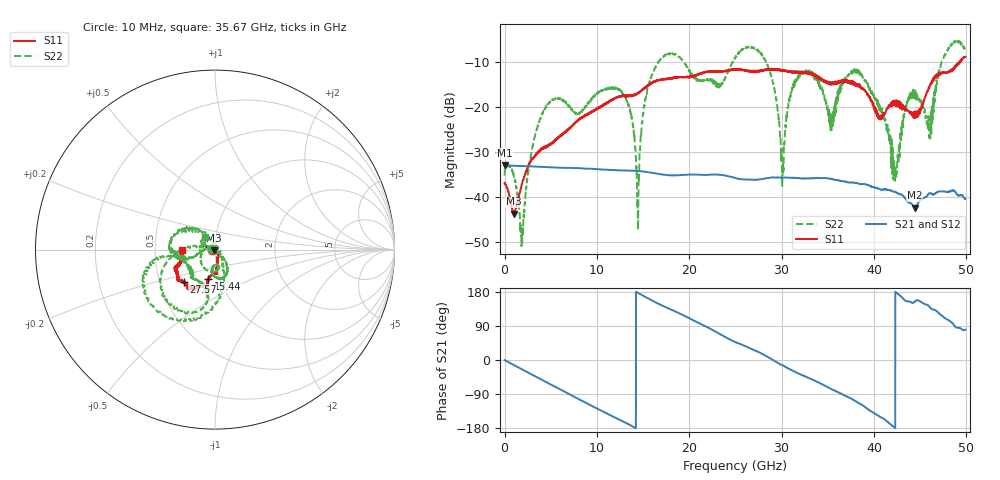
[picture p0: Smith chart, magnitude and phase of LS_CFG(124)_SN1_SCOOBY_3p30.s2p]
!Keysight Technologies,N5245B,MY58422026,A.13.80.08
!Date: Friday, March 20, 2020 00:06:09
!Correction: S11(Full 2 Port(1,2))
!S21(Full 2 Port(1,2))
!S12(Full 2 Port(1,2))
!S22(Full 2 Port(1,2))
!S2P File: Measurements: S11, S21, S12, S22:
# Hz S DB R 50.0
!freq dBS11 angS11 dBS21 angS21 dBS12 angS12 dBS22 angS22
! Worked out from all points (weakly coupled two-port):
!   4991 points, 10 MHz to 49.91 GHz, reference 50 ohm
!   highest |S21| = -32.99 dB at 10 MHz (marker M1); lowest = -42.5 dB at 44.42 GHz (marker M2)
!   lowest |S11| = -43.8 dB at 990 MHz (marker M3), VSWR 1.01, Z = 49.5 - j0.438 ohm
!   |S11| at or under -10 dB: start of sweep to 49.24 GHz; 49.29711 GHz to 49.33334 GHz (36.24 MHz wide, 0.0735 % of centre)
!   |S22| runs from -51.0 to -5.1 dB; largest |S21 - S12| = 0.00022
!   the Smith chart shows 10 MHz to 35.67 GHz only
!   S11 on the Smith chart (normalised r, x): 10 MHz: 0.97, -0.01; 15.44 GHz: 0.88, -0.30; 27.57 GHz: 0.66, -0.25; 35.67 GHz: 0.69, -0.01
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1e7  -36.94 -168.7  -32.99 -0.3  -32.98 -0.4  -35.30 176.8
9.9e8  -43.79 -136.8  -33.08 -13.0  -33.08 -13.0  -35.18 -121.0
1.9e9  -37.10 -65.0  -33.14 -24.8  -33.13 -24.7  -49.32 0.0
4.23e9  -29.26 -58.5  -33.35 -54.6  -33.34 -54.6  -20.86 -150.8
8.33e9  -22.50 -80.3  -33.67 -107.2  -33.67 -107.1  -20.98 -93.1
1.276e10  -17.55 -85.1  -34.12 -161.3  -34.12 -161.2  -16.79 -63.2
1.444e10  -16.92 -96.6  -34.25 177.3  -34.24 177.3  -46.16 -94.1
1.544e10  -15.42 -103.2  -34.51 164.0  -34.50 164.1  -16.41 174.1
1.665e10  -14.03 -102.2  -34.90 148.6  -34.89 148.7  -9.98 -157.4
2.496e10  -11.65 -124.9  -35.77 47.6  -35.76 47.7  -9.08 -167.8
2.757e10  -12.04 -134.4  -36.15 20.3  -36.13 20.4  -7.73 -109.8
3.011e10  -11.93 -143.6  -35.79 -13.7  -35.79 -13.6  -34.67 15.2
3.116e10  -12.09 -148.2  -35.78 -27.5  -35.78 -27.3  -15.60 140.3
3.328e10  -12.58 -157.7  -35.88 -51.3  -35.87 -51.0  -12.32 -175.2
3.567e10  -14.78 -178.5  -36.17 -79.9  -36.11 -79.5  -20.89 128.0
3.816e10  -15.32 175.4  -36.98 -110.7  -36.91 -111.0  -11.57 -174.7
4.16e10  -19.70 106.3  -38.48 -165.6  -38.49 -165.9  -25.63 67.7
4.233e10  -18.80 106.0  -38.96 179.9  -38.97 179.7  -33.70 164.4
4.442e10  -22.47 58.3  -42.45 153.8  -42.48 153.9  -17.80 -11.0
4.601e10  -15.69 6.5  -39.20 140.4  -39.21 140.3  -23.27 116.8
4.771e10  -12.26 7.1  -38.83 109.9  -38.82 110.0  -8.16 -80.0
4.991e10  -8.74 -12.6  -40.46 79.9  -40.48 79.7  -7.37 -14.7
